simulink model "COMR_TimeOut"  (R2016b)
settings: Solver=FixedStepDiscrete  StartTime=0.0  StopTime=10.0  FixedStep=0.01  RelTol=1e-3  EnableMultiTasking=on
undefined symbols (not defined in the file or in its folder): bin2dec, COMR_cntObcTmtDiag_CW, COMR_cntVcu2A3TmtDiag_CW, COMR_flgTmtCAB_C, COMR_numPackVcuMsg_C, COMR_tiBusoffDiagEna_C, COMR_tiCabMsgTmt_C, COMR_tiCSCMsgTmt_C, COMR_tiGWMsg050Tmt_C, COMR_tiGWMsgTmt_C, COMR_tiHv638MsgTmt_C, COMR_tiMcuMsgTmt_C, COMR_tiObcMsgTmt_C, COMR_tiPackVcuMsgTmt_C, COMR_tiPwrupDiagEna_C, COMR_tiTmtBase_C, COMR_tiVcuMsgTmt_C, COMR_UAESFltDiagDisbl_C
libraries: simulink x167
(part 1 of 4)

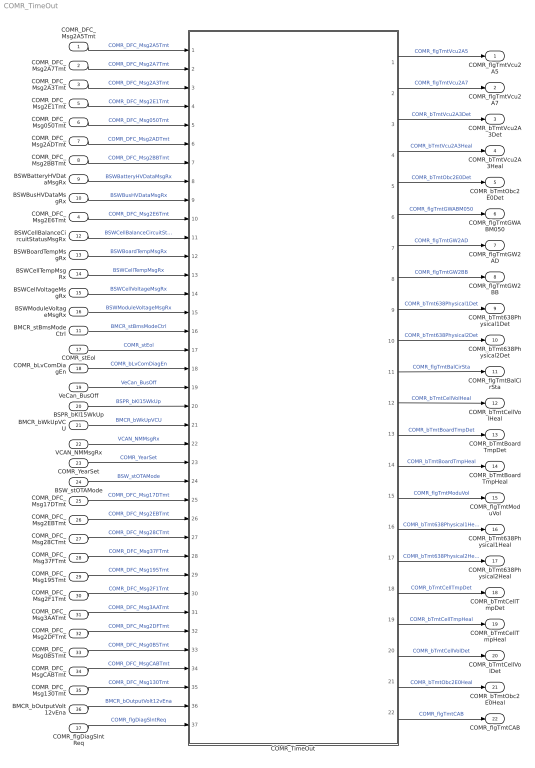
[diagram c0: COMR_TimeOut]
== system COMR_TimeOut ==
  COMR_DFC_Msg2A5Tmt : Inport
  COMR_DFC_Msg2A7Tmt : Inport  Port=2
  COMR_DFC_Msg2A3Tmt : Inport  Port=3
  COMR_DFC_Msg2E6Tmt : Inport  Port=4
  COMR_DFC_Msg2E1Tmt : Inport  Port=5
  COMR_DFC_Msg050Tmt : Inport  Port=6
  COMR_DFC_Msg2ADTmt : Inport  Port=7
  COMR_DFC_Msg2BBTmt : Inport  Port=8
  BSWBatteryHVDataMsgRx : Inport  Port=9
  BSWBusHVDataMsgRx : Inport  Port=10
  BMCR_stBmsModeCtrl : Inport  Port=11
  BSWCellBalanceCircuitStatusMsgRx : Inport  Port=12
  BSWBoardTempMsgRx : Inport  Port=13
  BSWCellTempMsgRx : Inport  Port=14
  BSWCellVoltageMsgRx : Inport  Port=15
  BSWModuleVoltageMsgRx : Inport  Port=16
  COMR_stEol : Inport  Port=17  OutDataTypeStr=boolean
  COMR_bLvComDiagEn : Inport  Port=18
  VeCan_BusOff : Inport  Port=19
  BSPR_bKl15WkUp : Inport  Port=20  OutDataTypeStr=boolean
  BMCR_bWkUpVCU : Inport  Port=21
  VCAN_NMMsgRx : Inport  Port=22
  COMR_YearSet : Inport  Port=23
  BSW_stOTAMode : Inport  Port=24  OutDataTypeStr=boolean
  COMR_DFC_Msg17DTmt : Inport  Port=25
  COMR_DFC_Msg2EBTmt : Inport  Port=26
  COMR_DFC_Msg28CTmt : Inport  Port=27
  COMR_DFC_Msg37FTmt : Inport  Port=28
  COMR_DFC_Msg195Tmt : Inport  Port=29
  COMR_DFC_Msg2F1Tmt : Inport  Port=30
  COMR_DFC_Msg3AATmt : Inport  Port=31
  COMR_DFC_Msg2DFTmt : Inport  Port=32
  COMR_DFC_Msg0B5Tmt : Inport  Port=33
  COMR_DFC_MsgCABTmt : Inport  Port=34
  COMR_DFC_Msg130Tmt : Inport  Port=35
  BMCR_bOutputVolt12vEna : Inport  Port=36
  COMR_flgDiagSlntReq : Inport  Port=37  OutDataTypeStr=boolean
  COMR_TimeOut : Subsystem
  COMR_flgTmtVcu2A5 : Outport
  COMR_flgTmtVcu2A7 : Outport  Port=2
  COMR_bTmtVcu2A3Det : Outport  Port=3
  COMR_bTmtVcu2A3Heal : Outport  Port=4
  COMR_bTmtObc2E0Det : Outport  Port=5
  COMR_flgTmtGWABM050 : Outport  Port=6
  COMR_flgTmtGW2AD : Outport  Port=7
  COMR_flgTmtGW2BB : Outport  Port=8
  COMR_bTmt638Physical1Det : Outport  Port=9
  COMR_bTmt638Physical2Det : Outport  Port=10
  COMR_flgTmtBalCirSta : Outport  Port=11
  COMR_bTmtCellVolHeal : Outport  Port=12
  COMR_bTmtBoardTmpDet : Outport  Port=13
  COMR_bTmtBoardTmpHeal : Outport  Port=14
  COMR_flgTmtModuVol : Outport  Port=15
  COMR_bTmt638Physical1Heal : Outport  Port=16
  COMR_bTmt638Physical2Heal : Outport  Port=17
  COMR_bTmtCellTmpDet : Outport  Port=18
  COMR_bTmtCellTmpHeal : Outport  Port=19
  COMR_bTmtCellVolDet : Outport  Port=20
  COMR_bTmtObc2E0Heal : Outport  Port=21
  COMR_flgTmtCAB : Outport  Port=22
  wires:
  COMR_DFC_Msg2A5Tmt/1 -> COMR_TimeOut/1(COMR_DFC_Msg2A5Tmt)  "COMR_DFC_Msg2A5Tmt"
  COMR_DFC_Msg2A7Tmt/1 -> COMR_TimeOut/2(COMR_DFC_Msg2A7Tmt)  "COMR_DFC_Msg2A7Tmt"
  COMR_DFC_Msg2A3Tmt/1 -> COMR_TimeOut/3(COMR_DFC_Msg2A3Tmt)  "COMR_DFC_Msg2A3Tmt"
  COMR_DFC_Msg2E6Tmt/1 -> COMR_TimeOut/10(COMR_DFC_Msg2E6Tmt)  "COMR_DFC_Msg2E6Tmt"
  COMR_DFC_Msg2E1Tmt/1 -> COMR_TimeOut/4(COMR_DFC_Msg2E1Tmt)  "COMR_DFC_Msg2E1Tmt"
  COMR_DFC_Msg050Tmt/1 -> COMR_TimeOut/5(COMR_DFC_Msg050Tmt)  "COMR_DFC_Msg050Tmt"
  COMR_DFC_Msg2ADTmt/1 -> COMR_TimeOut/6(COMR_DFC_Msg2ADTmt)  "COMR_DFC_Msg2ADTmt"
  COMR_DFC_Msg2BBTmt/1 -> COMR_TimeOut/7(COMR_DFC_Msg2BBTmt)  "COMR_DFC_Msg2BBTmt"
  BSWBatteryHVDataMsgRx/1 -> COMR_TimeOut/8(BSWBatteryHVDataMsgRx)  "BSWBatteryHVDataMsgRx"
  BSWBusHVDataMsgRx/1 -> COMR_TimeOut/9(BSWBusHVDataMsgRx)  "BSWBusHVDataMsgRx"
  COMR_TimeOut/1(COMR_flgTmtVcu2A5) -> COMR_flgTmtVcu2A5/1  "COMR_flgTmtVcu2A5"
  COMR_TimeOut/2(COMR_flgTmtVcu2A7) -> COMR_flgTmtVcu2A7/1  "COMR_flgTmtVcu2A7"
  COMR_TimeOut/3(COMR_bTmtVcu2A3Det) -> COMR_bTmtVcu2A3Det/1  "COMR_bTmtVcu2A3Det"
  COMR_TimeOut/4(COMR_bTmtVcu2A3Heal) -> COMR_bTmtVcu2A3Heal/1  "COMR_bTmtVcu2A3Heal"
  COMR_TimeOut/5(COMR_bTmtObc2E0Det) -> COMR_bTmtObc2E0Det/1  "COMR_bTmtObc2E0Det"
  COMR_TimeOut/6(COMR_flgTmtGWABM050) -> COMR_flgTmtGWABM050/1  "COMR_flgTmtGWABM050"
  COMR_TimeOut/7(COMR_flgTmtGW2AD) -> COMR_flgTmtGW2AD/1  "COMR_flgTmtGW2AD"
  COMR_TimeOut/8(COMR_flgTmtGW2BB) -> COMR_flgTmtGW2BB/1  "COMR_flgTmtGW2BB"
  COMR_TimeOut/9(COMR_bTmt638Physical1Det) -> COMR_bTmt638Physical1Det/1  "COMR_bTmt638Physical1Det"
  COMR_TimeOut/10(COMR_bTmt638Physical2Det) -> COMR_bTmt638Physical2Det/1  "COMR_bTmt638Physical2Det"
  BMCR_stBmsModeCtrl/1 -> COMR_TimeOut/16(BMCR_stBmsModeCtrl)  "BMCR_stBmsModeCtrl"
  BSWCellBalanceCircuitStatusMsgRx/1 -> COMR_TimeOut/11(BSWCellBalanceCircuitStatusMsgRx)  "BSWCellBalanceCircuitStatusMsgRx"
  COMR_TimeOut/12(COMR_bTmtCellVolHeal) -> COMR_bTmtCellVolHeal/1  "COMR_bTmtCellVolHeal"
  COMR_TimeOut/11(COMR_flgTmtBalCirSta) -> COMR_flgTmtBalCirSta/1  "COMR_flgTmtBalCirSta"
  COMR_TimeOut/13(COMR_bTmtBoardTmpDet) -> COMR_bTmtBoardTmpDet/1  "COMR_bTmtBoardTmpDet"
  COMR_TimeOut/14(COMR_bTmtBoardTmpHeal) -> COMR_bTmtBoardTmpHeal/1  "COMR_bTmtBoardTmpHeal"
  COMR_TimeOut/15(COMR_flgTmtModuVol) -> COMR_flgTmtModuVol/1  "COMR_flgTmtModuVol"
  BSWBoardTempMsgRx/1 -> COMR_TimeOut/12(BSWBoardTempMsgRx)  "BSWBoardTempMsgRx"
  BSWCellTempMsgRx/1 -> COMR_TimeOut/13(BSWCellTempMsgRx)  "BSWCellTempMsgRx"
  BSWCellVoltageMsgRx/1 -> COMR_TimeOut/14(BSWCellVoltageMsgRx)  "BSWCellVoltageMsgRx"
  BSWModuleVoltageMsgRx/1 -> COMR_TimeOut/15(BSWModuleVoltageMsgRx)  "BSWModuleVoltageMsgRx"
  COMR_TimeOut/16(COMR_bTmt638Physical1Heal) -> COMR_bTmt638Physical1Heal/1  "COMR_bTmt638Physical1Heal"
  COMR_TimeOut/17(COMR_bTmt638Physical2Heal) -> COMR_bTmt638Physical2Heal/1  "COMR_bTmt638Physical2Heal"
  COMR_TimeOut/18(COMR_bTmtCellTmpDet) -> COMR_bTmtCellTmpDet/1  "COMR_bTmtCellTmpDet"
  COMR_TimeOut/19(COMR_bTmtCellTmpHeal) -> COMR_bTmtCellTmpHeal/1  "COMR_bTmtCellTmpHeal"
  COMR_TimeOut/20(COMR_bTmtCellVolDet) -> COMR_bTmtCellVolDet/1  "COMR_bTmtCellVolDet"
  COMR_TimeOut/21(COMR_bTmtObc2E0Heal) -> COMR_bTmtObc2E0Heal/1  "COMR_bTmtObc2E0Heal"
  COMR_stEol/1 -> COMR_TimeOut/17(COMR_stEol)  "COMR_stEol"
  COMR_bLvComDiagEn/1 -> COMR_TimeOut/18(COMR_bLvComDiagEn)  "COMR_bLvComDiagEn"
  VeCan_BusOff/1 -> COMR_TimeOut/19(VeCan_BusOff)  "VeCan_BusOff"
  BSPR_bKl15WkUp/1 -> COMR_TimeOut/20(BSPR_bKl15WkUp)  "BSPR_bKl15WkUp"
  BMCR_bWkUpVCU/1 -> COMR_TimeOut/21(BMCR_bWkUpVCU)  "BMCR_bWkUpVCU"
  VCAN_NMMsgRx/1 -> COMR_TimeOut/22(VCAN_NMMsgRx)  "VCAN_NMMsgRx"
  COMR_YearSet/1 -> COMR_TimeOut/23(COMR_YearSet)  "COMR_YearSet"
  COMR_TimeOut/22(COMR_flgTmtCAB) -> COMR_flgTmtCAB/1  "COMR_flgTmtCAB"
  BSW_stOTAMode/1 -> COMR_TimeOut/24(BSW_stOTAMode)  "BSW_stOTAMode"
  COMR_DFC_Msg17DTmt/1 -> COMR_TimeOut/25(COMR_DFC_Msg17DTmt)  "COMR_DFC_Msg17DTmt"
  COMR_DFC_Msg130Tmt/1 -> COMR_TimeOut/35(COMR_DFC_Msg130Tmt)  "COMR_DFC_Msg130Tmt"
  COMR_DFC_Msg2EBTmt/1 -> COMR_TimeOut/26(COMR_DFC_Msg2EBTmt)  "COMR_DFC_Msg2EBTmt"
  COMR_DFC_Msg28CTmt/1 -> COMR_TimeOut/27(COMR_DFC_Msg28CTmt)  "COMR_DFC_Msg28CTmt"
  COMR_DFC_Msg37FTmt/1 -> COMR_TimeOut/28(COMR_DFC_Msg37FTmt)  "COMR_DFC_Msg37FTmt"
  COMR_DFC_Msg195Tmt/1 -> COMR_TimeOut/29(COMR_DFC_Msg195Tmt)  "COMR_DFC_Msg195Tmt"
  COMR_DFC_Msg2F1Tmt/1 -> COMR_TimeOut/30(COMR_DFC_Msg2F1Tmt)  "COMR_DFC_Msg2F1Tmt"
  COMR_DFC_Msg3AATmt/1 -> COMR_TimeOut/31(COMR_DFC_Msg3AATmt)  "COMR_DFC_Msg3AATmt"
  COMR_DFC_Msg2DFTmt/1 -> COMR_TimeOut/32(COMR_DFC_Msg2DFTmt)  "COMR_DFC_Msg2DFTmt"
  COMR_DFC_Msg0B5Tmt/1 -> COMR_TimeOut/33(COMR_DFC_Msg0B5Tmt)  "COMR_DFC_Msg0B5Tmt"
  COMR_DFC_MsgCABTmt/1 -> COMR_TimeOut/34(COMR_DFC_MsgCABTmt)  "COMR_DFC_MsgCABTmt"
  BMCR_bOutputVolt12vEna/1 -> COMR_TimeOut/36(BMCR_bOutputVolt12vEna)  "BMCR_bOutputVolt12vEna"
  COMR_flgDiagSlntReq/1 -> COMR_TimeOut/37(COMR_flgDiagSlntReq)  "COMR_flgDiagSlntReq"

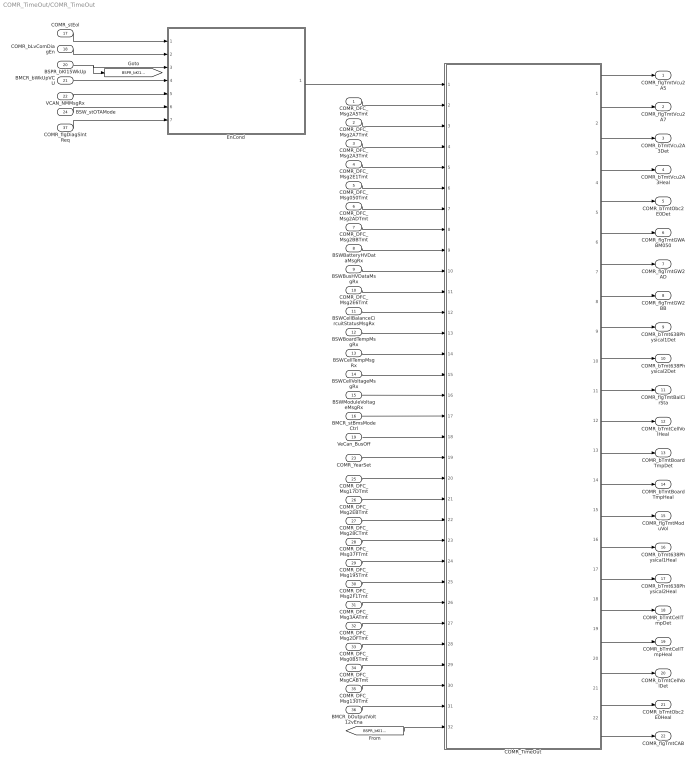
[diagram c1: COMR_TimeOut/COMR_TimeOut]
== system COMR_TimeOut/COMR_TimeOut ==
  COMR_DFC_Msg2A5Tmt : Inport
  COMR_DFC_Msg2A7Tmt : Inport  Port=2
  COMR_DFC_Msg2A3Tmt : Inport  Port=3
  COMR_DFC_Msg2E1Tmt : Inport  Port=4
  COMR_DFC_Msg050Tmt : Inport  Port=5
  COMR_DFC_Msg2ADTmt : Inport  Port=6
  COMR_DFC_Msg2BBTmt : Inport  Port=7
  BSWBatteryHVDataMsgRx : Inport  Port=8
  BSWBusHVDataMsgRx : Inport  Port=9
  COMR_DFC_Msg2E6Tmt : Inport  Port=10
  BSWCellBalanceCircuitStatusMsgRx : Inport  Port=11
  BSWBoardTempMsgRx : Inport  Port=12
  BSWCellTempMsgRx : Inport  Port=13
  BSWCellVoltageMsgRx : Inport  Port=14
  BSWModuleVoltageMsgRx : Inport  Port=15
  BMCR_stBmsModeCtrl : Inport  Port=16
  COMR_stEol : Inport  Port=17  OutDataTypeStr=boolean
  COMR_bLvComDiagEn : Inport  Port=18
  VeCan_BusOff : Inport  Port=19
  BSPR_bKl15WkUp : Inport  Port=20  OutDataTypeStr=boolean
  BMCR_bWkUpVCU : Inport  Port=21
  VCAN_NMMsgRx : Inport  Port=22
  COMR_YearSet : Inport  Port=23
  BSW_stOTAMode : Inport  Port=24  OutDataTypeStr=boolean
  COMR_DFC_Msg17DTmt : Inport  Port=25
  COMR_DFC_Msg2EBTmt : Inport  Port=26
  COMR_DFC_Msg28CTmt : Inport  Port=27
  COMR_DFC_Msg37FTmt : Inport  Port=28
  COMR_DFC_Msg195Tmt : Inport  Port=29
  COMR_DFC_Msg2F1Tmt : Inport  Port=30
  COMR_DFC_Msg3AATmt : Inport  Port=31
  COMR_DFC_Msg2DFTmt : Inport  Port=32
  COMR_DFC_Msg0B5Tmt : Inport  Port=33
  COMR_DFC_MsgCABTmt : Inport  Port=34
  COMR_DFC_Msg130Tmt : Inport  Port=35
  BMCR_bOutputVolt12vEna : Inport  Port=36
  COMR_flgDiagSlntReq : Inport  Port=37  OutDataTypeStr=boolean
  COMR_TimeOut : Subsystem
  EnCond : Subsystem
  COMR_flgTmtVcu2A5 : Outport
  COMR_flgTmtVcu2A7 : Outport  Port=2
  COMR_bTmtVcu2A3Det : Outport  Port=3
  COMR_bTmtVcu2A3Heal : Outport  Port=4
  COMR_bTmtObc2E0Det : Outport  Port=5
  COMR_flgTmtGWABM050 : Outport  Port=6
  COMR_flgTmtGW2AD : Outport  Port=7
  COMR_flgTmtGW2BB : Outport  Port=8
  COMR_bTmt638Physical1Det : Outport  Port=9
  COMR_bTmt638Physical2Det : Outport  Port=10
  COMR_flgTmtBalCirSta : Outport  Port=11
  COMR_bTmtCellVolHeal : Outport  Port=12
  COMR_bTmtBoardTmpDet : Outport  Port=13
  COMR_bTmtBoardTmpHeal : Outport  Port=14
  COMR_flgTmtModuVol : Outport  Port=15
  COMR_bTmt638Physical1Heal : Outport  Port=16
  COMR_bTmt638Physical2Heal : Outport  Port=17
  COMR_bTmtCellTmpDet : Outport  Port=18
  COMR_bTmtCellTmpHeal : Outport  Port=19
  COMR_bTmtCellVolDet : Outport  Port=20
  COMR_bTmtObc2E0Heal : Outport  Port=21
  COMR_flgTmtCAB : Outport  Port=22
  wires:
  COMR_DFC_Msg2A5Tmt/1 -> COMR_TimeOut/2(COMR_DFC_Msg2A5Tmt)
  COMR_DFC_Msg2A7Tmt/1 -> COMR_TimeOut/3(COMR_DFC_Msg2A7Tmt)
  COMR_DFC_Msg2A3Tmt/1 -> COMR_TimeOut/4(COMR_DFC_Msg2A3Tmt)
  COMR_DFC_Msg2E1Tmt/1 -> COMR_TimeOut/5(COMR_DFC_Msg2E1Tmt)
  COMR_DFC_Msg050Tmt/1 -> COMR_TimeOut/6(COMR_DFC_Msg050Tmt)
  COMR_DFC_Msg2ADTmt/1 -> COMR_TimeOut/7(COMR_DFC_Msg2ADTmt)
  COMR_DFC_Msg2BBTmt/1 -> COMR_TimeOut/8(COMR_DFC_Msg2BBTmt)
  BSWBatteryHVDataMsgRx/1 -> COMR_TimeOut/9(BSWBatteryHVDataMsgRx)
  BSWBusHVDataMsgRx/1 -> COMR_TimeOut/10(BSWBusHVDataMsgRx)
  COMR_DFC_Msg2E6Tmt/1 -> COMR_TimeOut/11(COMR_DFC_Msg2E6Tmt)
  BSWCellBalanceCircuitStatusMsgRx/1 -> COMR_TimeOut/12(BSWCellBalanceCircuitStatusMsgRx)
  BSWBoardTempMsgRx/1 -> COMR_TimeOut/13(BSWBoardTempMsgRx)
  BSWCellTempMsgRx/1 -> COMR_TimeOut/14(BSWCellTempMsgRx)
  BSWCellVoltageMsgRx/1 -> COMR_TimeOut/15(BSWCellVoltageMsgRx)
  BSWModuleVoltageMsgRx/1 -> COMR_TimeOut/16(BSWModuleVoltageMsgRx)
  BMCR_stBmsModeCtrl/1 -> COMR_TimeOut/17(BMCR_stBmsModeCtrl)
  COMR_TimeOut/1(COMR_flgTmtVcu2A5) -> COMR_flgTmtVcu2A5/1
  COMR_TimeOut/2(COMR_flgTmtVcu2A7) -> COMR_flgTmtVcu2A7/1
  COMR_TimeOut/3(COMR_bTmtVcu2A3Det) -> COMR_bTmtVcu2A3Det/1
  COMR_TimeOut/4(COMR_bTmtVcu2A3Heal) -> COMR_bTmtVcu2A3Heal/1
  COMR_TimeOut/5(COMR_bTmtObc2E0Det) -> COMR_bTmtObc2E0Det/1
  COMR_TimeOut/6(COMR_flgTmtGWABM050) -> COMR_flgTmtGWABM050/1
  COMR_TimeOut/7(COMR_flgTmtGW2AD) -> COMR_flgTmtGW2AD/1
  COMR_TimeOut/8(COMR_flgTmtGW2BB) -> COMR_flgTmtGW2BB/1
  COMR_TimeOut/9(COMR_bTmt638Physical1Det) -> COMR_bTmt638Physical1Det/1
  COMR_TimeOut/10(COMR_bTmt638Physical2Det) -> COMR_bTmt638Physical2Det/1
  COMR_TimeOut/11(COMR_flgTmtBalCirSta) -> COMR_flgTmtBalCirSta/1
  COMR_TimeOut/12(COMR_bTmtCellVolHeal) -> COMR_bTmtCellVolHeal/1
  COMR_TimeOut/13(COMR_bTmtBoardTmpDet) -> COMR_bTmtBoardTmpDet/1
  COMR_TimeOut/14(COMR_bTmtBoardTmpHeal) -> COMR_bTmtBoardTmpHeal/1
  COMR_TimeOut/15(COMR_flgTmtModuVol) -> COMR_flgTmtModuVol/1
  COMR_TimeOut/16(COMR_bTmt638Physical1Heal) -> COMR_bTmt638Physical1Heal/1
  COMR_TimeOut/17(COMR_bTmt638Physical2Heal) -> COMR_bTmt638Physical2Heal/1
  COMR_TimeOut/18(COMR_bTmtCellTmpDet) -> COMR_bTmtCellTmpDet/1
  COMR_TimeOut/19(COMR_bTmtCellTmpHeal) -> COMR_bTmtCellTmpHeal/1
  COMR_TimeOut/20(COMR_bTmtCellVolDet) -> COMR_bTmtCellVolDet/1
  COMR_TimeOut/21(COMR_bTmtObc2E0Heal) -> COMR_bTmtObc2E0Heal/1
  COMR_stEol/1 -> EnCond/1(COMR_stEol)
  EnCond/1(COMR_bTiOutChkEn) -> COMR_TimeOut/1(COMR_bTiOutChkEn)
  COMR_bLvComDiagEn/1 -> EnCond/2(COMR_bLvComDiagEn)
  VeCan_BusOff/1 -> COMR_TimeOut/18(VeCan_BusOff)
  BSPR_bKl15WkUp/1 -> EnCond/3(BSPR_bKl15WkUp), [BSPR_bKl15WkUp]
  BMCR_bWkUpVCU/1 -> EnCond/4(BMCR_bWkUpVCU)
  VCAN_NMMsgRx/1 -> EnCond/5(VCAN_NMMsgRx)
  COMR_YearSet/1 -> COMR_TimeOut/19(COMR_YearSet)
  COMR_TimeOut/22(COMR_flgTmtCAB) -> COMR_flgTmtCAB/1
  BSW_stOTAMode/1 -> EnCond/6(BSW_stOTAMode)
  COMR_DFC_Msg17DTmt/1 -> COMR_TimeOut/20(COMR_DFC_Msg17DTmt)
  COMR_DFC_Msg130Tmt/1 -> COMR_TimeOut/30(COMR_DFC_Msg130Tmt)
  COMR_DFC_Msg2EBTmt/1 -> COMR_TimeOut/21(COMR_DFC_Msg2EBTmt)
  COMR_DFC_Msg28CTmt/1 -> COMR_TimeOut/22(COMR_DFC_Msg28CTmt)
  COMR_DFC_Msg37FTmt/1 -> COMR_TimeOut/23(COMR_DFC_Msg37FTmt)
  COMR_DFC_Msg195Tmt/1 -> COMR_TimeOut/24(COMR_DFC_Msg195Tmt)
  COMR_DFC_Msg2F1Tmt/1 -> COMR_TimeOut/25(COMR_DFC_Msg2F1Tmt)
  COMR_DFC_Msg3AATmt/1 -> COMR_TimeOut/26(COMR_DFC_Msg3AATmt)
  COMR_DFC_Msg2DFTmt/1 -> COMR_TimeOut/27(COMR_DFC_Msg2DFTmt)
  COMR_DFC_Msg0B5Tmt/1 -> COMR_TimeOut/28(COMR_DFC_Msg0B5Tmt)
  COMR_DFC_MsgCABTmt/1 -> COMR_TimeOut/29(COMR_DFC_MsgCABTmt)
  BMCR_bOutputVolt12vEna/1 -> COMR_TimeOut/31(BMCR_bOutputVolt12vEna)
  COMR_flgDiagSlntReq/1 -> EnCond/7(COMR_flgDiagSlntReq)
  [BSPR_bKl15WkUp] -> COMR_TimeOut/32(BSPR_bKl15WkUp)

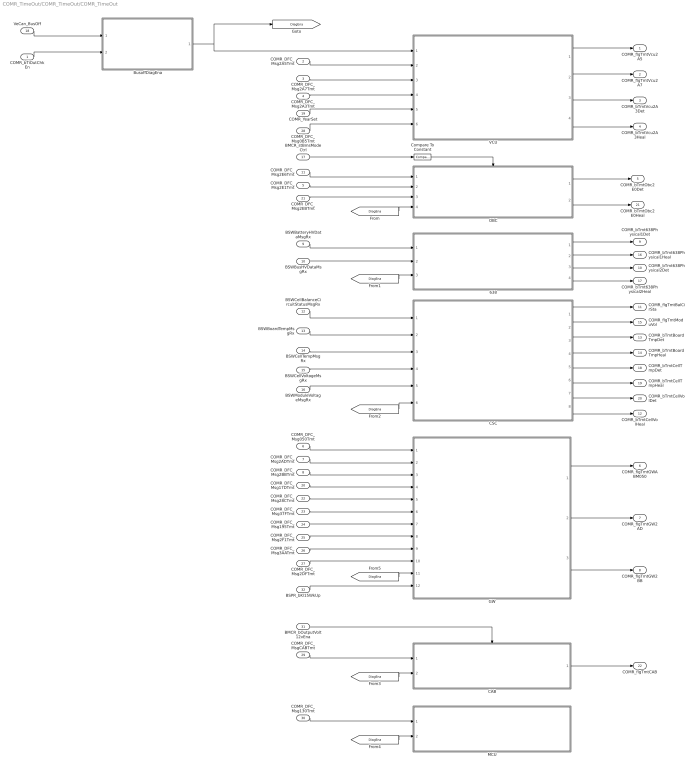
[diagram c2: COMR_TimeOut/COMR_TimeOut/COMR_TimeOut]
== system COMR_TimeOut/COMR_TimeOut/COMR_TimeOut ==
  COMR_bTiOutChkEn : Inport
  COMR_DFC_Msg2A5Tmt : Inport  Port=2
  COMR_DFC_Msg2A7Tmt : Inport  Port=3
  COMR_DFC_Msg2A3Tmt : Inport  Port=4
  COMR_DFC_Msg2E1Tmt : Inport  Port=5
  COMR_DFC_Msg050Tmt : Inport  Port=6
  COMR_DFC_Msg2ADTmt : Inport  Port=7
  COMR_DFC_Msg2BBTmt : Inport  Port=8
  BSWBatteryHVDataMsgRx : Inport  Port=9
  BSWBusHVDataMsgRx : Inport  Port=10
  COMR_DFC_Msg2E6Tmt : Inport  Port=11
  BSWCellBalanceCircuitStatusMsgRx : Inport  Port=12
  BSWBoardTempMsgRx : Inport  Port=13
  BSWCellTempMsgRx : Inport  Port=14
  BSWCellVoltageMsgRx : Inport  Port=15
  BSWModuleVoltageMsgRx : Inport  Port=16
  BMCR_stBmsModeCtrl : Inport  Port=17
  VeCan_BusOff : Inport  Port=18
  COMR_YearSet : Inport  Port=19
  COMR_DFC_Msg17DTmt : Inport  Port=20
  COMR_DFC_Msg2EBTmt : Inport  Port=21
  COMR_DFC_Msg28CTmt : Inport  Port=22
  COMR_DFC_Msg37FTmt : Inport  Port=23
  COMR_DFC_Msg195Tmt : Inport  Port=24
  COMR_DFC_Msg2F1Tmt : Inport  Port=25
  COMR_DFC_Msg3AATmt : Inport  Port=26
  COMR_DFC_Msg2DFTmt : Inport  Port=27
  COMR_DFC_Msg0B5Tmt : Inport  Port=28
  COMR_DFC_MsgCABTmt : Inport  Port=29
  COMR_DFC_Msg130Tmt : Inport  Port=30
  BMCR_bOutputVolt12vEna : Inport  Port=31
  BSPR_bKl15WkUp : Inport  Port=32  OutDataTypeStr=boolean
  638 : Subsystem
  BusoffDiagEna : Subsystem
  CAB : Subsystem
  CSC : Subsystem
  Compare To Constant : simulink/Logic and Bit Operations/Compare To Constant  relop===  const=6  OutDataTypeStr=boolean
  GW : Subsystem
  MCU : Subsystem
  OBC : Subsystem
  VCU : Subsystem
  COMR_flgTmtVcu2A5 : Outport  InitialOutput=[0]
  COMR_flgTmtVcu2A7 : Outport  Port=2  InitialOutput=[0]
  COMR_bTmtVcu2A3Det : Outport  Port=3  InitialOutput=[0]
  COMR_bTmtVcu2A3Heal : Outport  Port=4  InitialOutput=[0]
  COMR_bTmtObc2E0Det : Outport  Port=5  InitialOutput=[0]
  COMR_flgTmtGWABM050 : Outport  Port=6
  COMR_flgTmtGW2AD : Outport  Port=7
  COMR_flgTmtGW2BB : Outport  Port=8
  COMR_bTmt638Physical1Det : Outport  Port=9  InitialOutput=[0]
  COMR_bTmt638Physical2Det : Outport  Port=10
  COMR_flgTmtBalCirSta : Outport  Port=11  InitialOutput=[0]
  COMR_bTmtCellVolHeal : Outport  Port=12
  COMR_bTmtBoardTmpDet : Outport  Port=13
  COMR_bTmtBoardTmpHeal : Outport  Port=14
  COMR_flgTmtModuVol : Outport  Port=15  InitialOutput=[0]
  COMR_bTmt638Physical1Heal : Outport  Port=16
  COMR_bTmt638Physical2Heal : Outport  Port=17
  COMR_bTmtCellTmpDet : Outport  Port=18
  COMR_bTmtCellTmpHeal : Outport  Port=19
  COMR_bTmtCellVolDet : Outport  Port=20
  COMR_bTmtObc2E0Heal : Outport  Port=21  InitialOutput=[0]
  COMR_flgTmtCAB : Outport  Port=22
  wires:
  BSWBoardTempMsgRx/1 -> CSC/2(BSWBoardTempMsgRx)
  COMR_DFC_Msg2A3Tmt/1 -> VCU/4(COMR_DFC_Msg2A3Tmt)
  COMR_DFC_Msg2A7Tmt/1 -> VCU/3(COMR_DFC_Msg2A7Tmt)
  638/4(COMR_bTmt638Physical2Heal) -> COMR_bTmt638Physical2Heal/1
  COMR_DFC_Msg2A5Tmt/1 -> VCU/2(COMR_DFC_Msg2A5Tmt)
  CSC/2(COMR_flgTmtModuVol) -> COMR_flgTmtModuVol/1
  CSC/3(COMR_bTmtBoardTmpDet) -> COMR_bTmtBoardTmpDet/1
  CSC/4(COMR_bTmtBoardTmpHeal) -> COMR_bTmtBoardTmpHeal/1
  CSC/8(COMR_bTmtCellVolHeal) -> COMR_bTmtCellVolHeal/1
  BSWCellBalanceCircuitStatusMsgRx/1 -> CSC/1(BSWCellBalanceCircuitStatusMsgRx)
  CSC/1(COMR_flgTmtBalCirSta) -> COMR_flgTmtBalCirSta/1
  638/3(COMR_bTmt638Physical2Det) -> COMR_bTmt638Physical2Det/1
  BSWBusHVDataMsgRx/1 -> 638/2(BSWBusHVDataMsgRx)
  638/1(COMR_bTmt638Physical1Det) -> COMR_bTmt638Physical1Det/1
  BSWBatteryHVDataMsgRx/1 -> 638/1(BSWBatteryHVDataMsgRx)
  GW/2(COMR_flgTmtGW2AD) -> COMR_flgTmtGW2AD/1
  GW/3(COMR_flgTmtGW2BB) -> COMR_flgTmtGW2BB/1
  GW/1(COMR_flgTmtGWABM050) -> COMR_flgTmtGWABM050/1
  COMR_DFC_Msg2ADTmt/1 -> GW/2(COMR_DFC_Msg2ADTmt)
  COMR_DFC_Msg2BBTmt/1 -> GW/3(COMR_DFC_Msg2BBTmt)
  638/2(COMR_bTmt638Physical1Heal) -> COMR_bTmt638Physical1Heal/1
  BMCR_stBmsModeCtrl/1 -> Compare To Constant/1
  BSWModuleVoltageMsgRx/1 -> CSC/5(BSWModuleVoltageMsgRx)
  BSWCellTempMsgRx/1 -> CSC/3(BSWCellTempMsgRx)
  BSWCellVoltageMsgRx/1 -> CSC/4(BSWCellVoltageMsgRx)
  OBC/1(COMR_bTmtObc2E6Det) -> COMR_bTmtObc2E0Det/1
  COMR_DFC_Msg050Tmt/1 -> GW/1(COMR_DFC_Msg050Tmt)
  COMR_DFC_Msg2E6Tmt/1 -> OBC/1(COMR_DFC_Msg2E6Tmt)
  VCU/4(COMR_bTmtVcu2A3Heal) -> COMR_bTmtVcu2A3Heal/1
  VCU/3(COMR_bTmtVcu2A3Det) -> COMR_bTmtVcu2A3Det/1
  COMR_DFC_Msg2E1Tmt/1 -> OBC/2(COMR_DFC_Msg2E1Tmt)
  VCU/1(COMR_flgTmtVcu2A5) -> COMR_flgTmtVcu2A5/1
  VCU/2(COMR_flgTmtVcu2A7) -> COMR_flgTmtVcu2A7/1
  CSC/5(COMR_bTmtCellTmpDet) -> COMR_bTmtCellTmpDet/1
  OBC/2(COMR_bTmtObc2E6Heal) -> COMR_bTmtObc2E0Heal/1
  CSC/7(COMR_bTmtCellVolDet) -> COMR_bTmtCellVolDet/1
  CSC/6(COMR_bTmtCellTmpHeal) -> COMR_bTmtCellTmpHeal/1
  Compare To Constant/1 -> OBC/Enable
  [DiagEna] -> OBC/4(DiagEna)
  [DiagEna] -> 638/3(DiagEna)
  [DiagEna] -> CSC/6(DiagEna)
  VeCan_BusOff/1 -> BusoffDiagEna/1(VeCan_BusOff)
  BusoffDiagEna/1(DiagEna) -> [DiagEna], VCU/1(DiagEna)
  COMR_YearSet/1 -> VCU/5(COMR_YearSet)
  CAB/1(COMR_flgTmtCAB) -> COMR_flgTmtCAB/1
  COMR_DFC_Msg0B5Tmt/1 -> VCU/6(COMR_DFC_Msg0B5Tmt)
  COMR_DFC_Msg2EBTmt/1 -> OBC/3(COMR_DFC_Msg2EBTmt)
  COMR_DFC_MsgCABTmt/1 -> CAB/1(COMR_DFC_MsgCABTmt)
  [DiagEna] -> CAB/2(DiagEna)
  [DiagEna] -> MCU/2(DiagEna)
  COMR_DFC_Msg130Tmt/1 -> MCU/1(COMR_DFC_Msg130Tmt)
  COMR_DFC_Msg17DTmt/1 -> GW/4(COMR_DFC_Msg17DTmt)
  COMR_DFC_Msg28CTmt/1 -> GW/5(COMR_DFC_Msg28CTmt)
  COMR_DFC_Msg37FTmt/1 -> GW/6(COMR_DFC_Msg37FTmt)
  COMR_DFC_Msg195Tmt/1 -> GW/7(COMR_DFC_Msg195Tmt)
  COMR_DFC_Msg2F1Tmt/1 -> GW/8(COMR_DFC_Msg2F1Tmt)
  COMR_DFC_Msg3AATmt/1 -> GW/9(COMR_DFC_Msg3AATmt)
  COMR_DFC_Msg2DFTmt/1 -> GW/10(COMR_DFC_Msg2DFTmt)
  [DiagEna] -> GW/11(DiagEna)
  BMCR_bOutputVolt12vEna/1 -> CAB/Enable
  COMR_bTiOutChkEn/1 -> BusoffDiagEna/2(COMR_bTiOutChkEn)
  BSPR_bKl15WkUp/1 -> GW/12(BSPR_bKl15WkUp)

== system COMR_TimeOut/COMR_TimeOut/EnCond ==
  COMR_stEol : Inport  OutDataTypeStr=boolean
  COMR_bLvComDiagEn : Inport  Port=2
  BSPR_bKl15WkUp : Inport  Port=3  OutDataTypeStr=boolean
  BMCR_bWkUpVCU : Inport  Port=4
  VCAN_NMMsgRx : Inport  Port=5
  BSW_stOTAMode : Inport  Port=6  OutDataTypeStr=boolean
  COMR_flgDiagSlntReq : Inport  Port=7  OutDataTypeStr=boolean
  Constant1 : Constant  Value=COMR_tiPwrupDiagEna_C
  Logical Operator : Logic  AllPortsSameDT=off  OutDataTypeStr=boolean
  Logical Operator1 : Logic  Operator=OR  Inputs=3  AllPortsSameDT=off  OutDataTypeStr=boolean
  Logical Operator2 : Logic  Operator=NOT  AllPortsSameDT=off  OutDataTypeStr=boolean
  Logical Operator3 : Logic  Inputs=4  AllPortsSameDT=off  OutDataTypeStr=boolean
  Logical Operator4 : Logic  Operator=NOT  AllPortsSameDT=off  OutDataTypeStr=boolean
  Logical Operator5 : Logic  Operator=NOT  AllPortsSameDT=off  OutDataTypeStr=boolean
  TONV_10msTimeDebounce : Subsystem  TreatAsAtomicUnit=on  RTWFcnName=TONV_10msTimeDebounce  RTWFileName=SrvLib
  COMR_bTiOutChkEn : Outport
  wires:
  Constant1/1 -> TONV_10msTimeDebounce/2(T)
  Logical Operator/1 -> COMR_bTiOutChkEn/1  "COMR_bTiOutChkEn"
  COMR_stEol/1 -> Logical Operator2/1
  TONV_10msTimeDebounce/1(y) -> Logical Operator/1
  COMR_bLvComDiagEn/1 -> Logical Operator/2
  BSPR_bKl15WkUp/1 -> Logical Operator1/1
  BMCR_bWkUpVCU/1 -> Logical Operator1/2
  VCAN_NMMsgRx/1 -> Logical Operator1/3
  Logical Operator2/1 -> Logical Operator3/2
  Logical Operator1/1 -> Logical Operator3/1
  Logical Operator3/1 -> TONV_10msTimeDebounce/1(u)
  Logical Operator4/1 -> Logical Operator3/3
  BSW_stOTAMode/1 -> Logical Operator4/1
  COMR_flgDiagSlntReq/1 -> Logical Operator5/1
  Logical Operator5/1 -> Logical Operator3/4

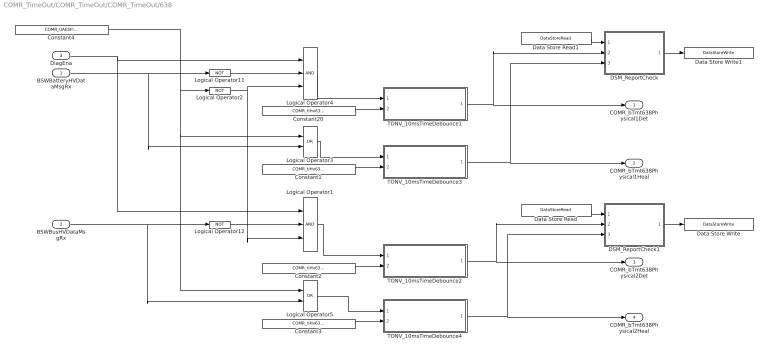
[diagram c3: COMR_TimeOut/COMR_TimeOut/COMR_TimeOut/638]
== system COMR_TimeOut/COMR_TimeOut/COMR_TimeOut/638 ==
  BSWBatteryHVDataMsgRx : Inport
  BSWBusHVDataMsgRx : Inport  Port=2
  DiagEna : Inport  Port=3
  Constant{1..3,20} (4 alike) : Constant  Value=COMR_tiHv638MsgTmt_C
  Constant4 : Constant  Value=COMR_UAESFltDiagDisbl_C
  DSM_ReportCheck : Subsystem  TreatAsAtomicUnit=on  RTWFcnName=DSM_ReportCheck  RTWFileName=SrvLib
  DSM_ReportCheck1 : Subsystem  TreatAsAtomicUnit=on  RTWFcnName=DSM_ReportCheck  RTWFileName=SrvLib
  Data Store Read : DataStoreRead  DataStoreName=DFC_BusHVMsgTmt
  Data Store Read1 : DataStoreRead  DataStoreName=DFC_BattHVMsgTmt
  Data Store Write : DataStoreWrite  DataStoreName=DFC_BusHVMsgTmt
  Data Store Write1 : DataStoreWrite  DataStoreName=DFC_BattHVMsgTmt
  Logical Operator1 : Logic  Inputs=3  AllPortsSameDT=off  OutDataTypeStr=boolean
  Logical Operator11 : Logic  Operator=NOT  AllPortsSameDT=off  OutDataTypeStr=boolean
  Logical Operator12 : Logic  Operator=NOT  AllPortsSameDT=off  OutDataTypeStr=boolean
  Logical Operator2 : Logic  Operator=NOT  AllPortsSameDT=off  OutDataTypeStr=boolean
  Logical Operator3 : Logic  Operator=OR  AllPortsSameDT=off  OutDataTypeStr=boolean
  Logical Operator4 : Logic  Inputs=3  AllPortsSameDT=off  OutDataTypeStr=boolean
  Logical Operator5 : Logic  Operator=OR  AllPortsSameDT=off  OutDataTypeStr=boolean
  TONV_10msTimeDebounce1 : Subsystem  TreatAsAtomicUnit=on  RTWFcnName=TONV_10msTimeDebounce  RTWFileName=SrvLib
  TONV_10msTimeDebounce2 : Subsystem  TreatAsAtomicUnit=on  RTWFcnName=TONV_10msTimeDebounce  RTWFileName=SrvLib
  TONV_10msTimeDebounce3 : Subsystem  TreatAsAtomicUnit=on  RTWFcnName=TONV_10msTimeDebounce  RTWFileName=SrvLib
  TONV_10msTimeDebounce4 : Subsystem  TreatAsAtomicUnit=on  RTWFcnName=TONV_10msTimeDebounce  RTWFileName=SrvLib
  COMR_bTmt638Physical1Det : Outport  InitialOutput=[0]
  COMR_bTmt638Physical1Heal : Outport  Port=2  InitialOutput=[0]
  COMR_bTmt638Physical2Det : Outport  Port=3  InitialOutput=[0]
  COMR_bTmt638Physical2Heal : Outport  Port=4  InitialOutput=[0]
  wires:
  TONV_10msTimeDebounce1/1(y) -> DSM_ReportCheck/2(Err), COMR_bTmt638Physical1Det/1
  Constant2/1 -> TONV_10msTimeDebounce2/2(T)
  Logical Operator11/1 -> Logical Operator4/2
  Constant20/1 -> TONV_10msTimeDebounce1/2(T)
  TONV_10msTimeDebounce3/1(y) -> DSM_ReportCheck/3(Heal), COMR_bTmt638Physical1Heal/1
  Constant1/1 -> TONV_10msTimeDebounce3/2(T)
  Constant3/1 -> TONV_10msTimeDebounce4/2(T)
  TONV_10msTimeDebounce2/1(y) -> DSM_ReportCheck1/2(Err), COMR_bTmt638Physical2Det/1
  TONV_10msTimeDebounce4/1(y) -> DSM_ReportCheck1/3(Heal), COMR_bTmt638Physical2Heal/1
  DSM_ReportCheck1/1(Dfc_id) -> Data Store Write/1
  Data Store Read/1 -> DSM_ReportCheck1/1(Dfc_id_nv)
  Data Store Read1/1 -> DSM_ReportCheck/1(Dfc_id_nv)
  DSM_ReportCheck/1(Dfc_id) -> Data Store Write1/1
  BSWBatteryHVDataMsgRx/1 -> Logical Operator3/2, Logical Operator11/1
  BSWBusHVDataMsgRx/1 -> Logical Operator12/1, Logical Operator5/2
  DiagEna/1 -> Logical Operator4/1, Logical Operator1/1
  Logical Operator1/1 -> TONV_10msTimeDebounce2/1(u)
  Logical Operator4/1 -> TONV_10msTimeDebounce1/1(u)
  Logical Operator12/1 -> Logical Operator1/2
  Constant4/1 -> Logical Operator5/1, Logical Operator3/1, Logical Operator2/1
  Logical Operator2/1 -> Logical Operator4/3, Logical Operator1/3
  Logical Operator3/1 -> TONV_10msTimeDebounce3/1(u)
  Logical Operator5/1 -> TONV_10msTimeDebounce4/1(u)

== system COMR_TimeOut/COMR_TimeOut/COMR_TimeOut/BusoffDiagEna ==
  VeCan_BusOff : Inport
  COMR_bTiOutChkEn : Inport  Port=2
  Constant10 : Constant  Value=COMR_UAESFltDiagDisbl_C
  Constant8 : Constant  Value=0  OutDataTypeStr=boolean
  EdgeFalling : Subsystem  TreatAsAtomicUnit=on  RTWFcnName=EdgeFalling  RTWFileName=SrvLib
  Logical Operator : Logic  Operator=NOT  AllPortsSameDT=off  OutDataTypeStr=boolean
  Logical Operator1 : Logic  AllPortsSameDT=off  OutDataTypeStr=boolean
  Logical Operator2 : Logic  AllPortsSameDT=off  OutDataTypeStr=boolean
  StateRetention2 : Subsystem
  Switch : Switch  Criteria=u2 ~= 0
  DiagEna : Outport
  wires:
  VeCan_BusOff/1 -> EdgeFalling/1(u), Logical Operator/1
  StateRetention2/1(_Out) -> Logical Operator1/1
  EdgeFalling/1(y) -> StateRetention2/1(u)
  Constant8/1 -> StateRetention2/2(clc)
  Logical Operator/1 -> Logical Operator1/2
  Logical Operator1/1 -> Switch/3
  Constant10/1 -> Switch/1, Switch/2
  Switch/1 -> Logical Operator2/1
  Logical Operator2/1 -> DiagEna/1
  COMR_bTiOutChkEn/1 -> Logical Operator2/2

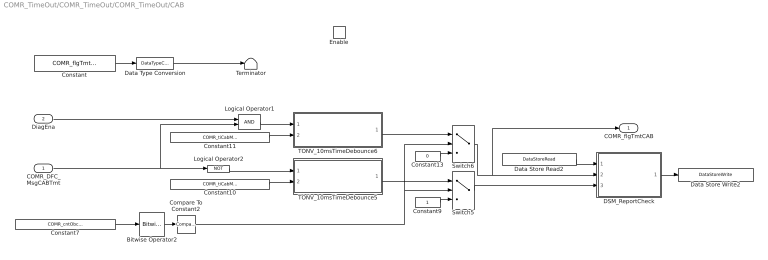
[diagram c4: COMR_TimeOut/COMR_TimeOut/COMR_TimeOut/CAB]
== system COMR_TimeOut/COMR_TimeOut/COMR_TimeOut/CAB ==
  COMR_DFC_MsgCABTmt : Inport
  DiagEna : Inport  Port=2
  Enable : EnablePort  StatesWhenEnabling=reset
  Bitwise Operator2 : simulink/Logic and Bit Operations/Bitwise Operator  logicop=AND  UseBitMask=on  BitMask=bin2dec('00010000')  BitMaskRealWorld=Stored Integer
  Compare To Constant2 : simulink/Logic and Bit Operations/Compare To Constant  relop===  const=16  OutDataTypeStr=boolean
  Constant : Constant  Value=COMR_flgTmtCAB_C
  Constant10 : Constant  Value=COMR_tiCabMsgTmt_C
  Constant11 : Constant  Value=COMR_tiCabMsgTmt_C
  Constant13 : Constant  Value=0  OutDataTypeStr=boolean
  Constant7 : Constant  Value=COMR_cntObcTmtDiag_CW
  Constant9 : Constant  OutDataTypeStr=boolean
  DSM_ReportCheck : Subsystem  TreatAsAtomicUnit=on  RTWFcnName=DSM_ReportCheck  RTWFileName=SrvLib
  Data Store Read2 : DataStoreRead  DataStoreName=DFC_MsgCABTmt
  Data Store Write2 : DataStoreWrite  DataStoreName=DFC_MsgCABTmt
  Data Type Conversion : DataTypeConversion  OutDataTypeStr=boolean
  Logical Operator1 : Logic  AllPortsSameDT=off  OutDataTypeStr=boolean
  Logical Operator2 : Logic  Operator=NOT  AllPortsSameDT=off  OutDataTypeStr=boolean
  Switch5 : Switch  Criteria=u2 > Threshold
  Switch6 : Switch  Criteria=u2 > Threshold
  TONV_10msTimeDebounce5 : Subsystem  TreatAsAtomicUnit=on  RTWFcnName=TONV_10msTimeDebounce  RTWFileName=SrvLib
  TONV_10msTimeDebounce6 : Subsystem  TreatAsAtomicUnit=on  RTWFcnName=TONV_10msTimeDebounce  RTWFileName=SrvLib
  Terminator : Terminator
  COMR_flgTmtCAB : Outport
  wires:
  Constant/1 -> Data Type Conversion/1
  Data Type Conversion/1 -> Terminator/1
  Compare To Constant2/1 -> Switch5/2, Switch6/2
  Constant7/1 -> Bitwise Operator2/1
  Bitwise Operator2/1 -> Compare To Constant2/1
  DiagEna/1 -> Logical Operator1/1
  Constant11/1 -> TONV_10msTimeDebounce6/2(T)
  DSM_ReportCheck/1(Dfc_id) -> Data Store Write2/1
  Constant10/1 -> TONV_10msTimeDebounce5/2(T)
  Constant13/1 -> Switch6/3
  Constant9/1 -> Switch5/3
  TONV_10msTimeDebounce6/1(y) -> Switch6/1
  TONV_10msTimeDebounce5/1(y) -> Switch5/1
  Switch5/1 -> DSM_ReportCheck/3(Heal)
  Data Store Read2/1 -> DSM_ReportCheck/1(Dfc_id_nv)
  Switch6/1 -> DSM_ReportCheck/2(Err), COMR_flgTmtCAB/1
  COMR_DFC_MsgCABTmt/1 -> Logical Operator1/2, Logical Operator2/1
  Logical Operator1/1 -> TONV_10msTimeDebounce6/1(u)
  Logical Operator2/1 -> TONV_10msTimeDebounce5/1(u)

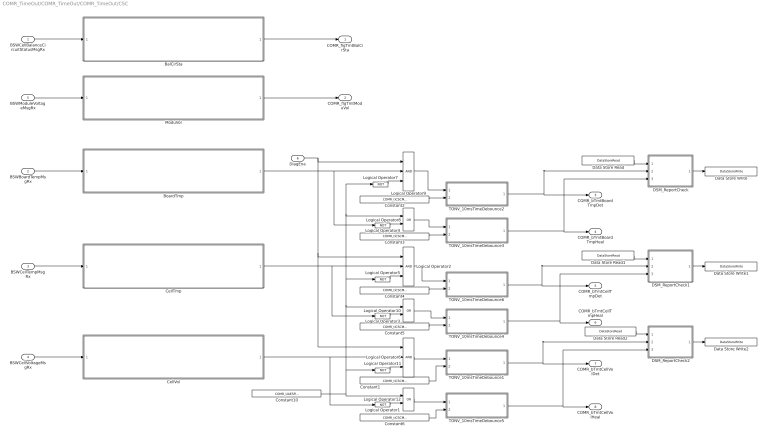
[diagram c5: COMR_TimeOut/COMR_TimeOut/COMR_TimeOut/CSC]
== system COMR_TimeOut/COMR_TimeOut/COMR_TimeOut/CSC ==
  BSWCellBalanceCircuitStatusMsgRx : Inport
  BSWBoardTempMsgRx : Inport  Port=2
  BSWCellTempMsgRx : Inport  Port=3
  BSWCellVoltageMsgRx : Inport  Port=4
  BSWModuleVoltageMsgRx : Inport  Port=5
  DiagEna : Inport  Port=6
  BalCirSta : Stateflow chart  TreatAsAtomicUnit=on
  BoardTmp : Stateflow chart  TreatAsAtomicUnit=on
  CellTmp : Stateflow chart  TreatAsAtomicUnit=on
  CellVol : Stateflow chart  TreatAsAtomicUnit=on
  Constant{1..6} (6 alike) : Constant  Value=COMR_tiCSCMsgTmt_C
  Constant10 : Constant  Value=COMR_UAESFltDiagDisbl_C
  DSM_ReportCheck : Subsystem  TreatAsAtomicUnit=on  RTWFcnName=DSM_ReportCheck  RTWFileName=SrvLib
  DSM_ReportCheck1 : Subsystem  TreatAsAtomicUnit=on  RTWFcnName=DSM_ReportCheck  RTWFileName=SrvLib
  DSM_ReportCheck2 : Subsystem  TreatAsAtomicUnit=on  RTWFcnName=DSM_ReportCheck  RTWFileName=SrvLib
  Data Store Read : DataStoreRead  DataStoreName=DFC_BoardTempTmt
  Data Store Read1 : DataStoreRead  DataStoreName=DFC_CellTempTmt
  Data Store Read2 : DataStoreRead  DataStoreName=DFC_CellVoltTmt
  Data Store Write : DataStoreWrite  DataStoreName=DFC_BoardTempTmt
  Data Store Write1 : DataStoreWrite  DataStoreName=DFC_CellTempTmt
  Data Store Write2 : DataStoreWrite  DataStoreName=DFC_CellVoltTmt
  Logical Operator{1,3..5,7,11} (6 alike) : Logic  Operator=NOT  AllPortsSameDT=off  OutDataTypeStr=boolean
  Logical Operator10 : Logic  Operator=OR  AllPortsSameDT=off  OutDataTypeStr=boolean
  Logical Operator12 : Logic  Operator=OR  AllPortsSameDT=off  OutDataTypeStr=boolean
  Logical Operator2 : Logic  Inputs=3  AllPortsSameDT=off  OutDataTypeStr=boolean
  Logical Operator6 : Logic  Inputs=3  AllPortsSameDT=off  OutDataTypeStr=boolean
  Logical Operator8 : Logic  Operator=OR  AllPortsSameDT=off  OutDataTypeStr=boolean
  Logical Operator9 : Logic  Inputs=3  AllPortsSameDT=off  OutDataTypeStr=boolean
  ModuVol : Stateflow chart  TreatAsAtomicUnit=on
  TONV_10msTimeDebounce1 : Subsystem  TreatAsAtomicUnit=on  RTWFcnName=TONV_10msTimeDebounce  RTWFileName=SrvLib
  TONV_10msTimeDebounce2 : Subsystem  TreatAsAtomicUnit=on  RTWFcnName=TONV_10msTimeDebounce  RTWFileName=SrvLib
  TONV_10msTimeDebounce3 : Subsystem  TreatAsAtomicUnit=on  RTWFcnName=TONV_10msTimeDebounce  RTWFileName=SrvLib
  TONV_10msTimeDebounce4 : Subsystem  TreatAsAtomicUnit=on  RTWFcnName=TONV_10msTimeDebounce  RTWFileName=SrvLib
  TONV_10msTimeDebounce5 : Subsystem  TreatAsAtomicUnit=on  RTWFcnName=TONV_10msTimeDebounce  RTWFileName=SrvLib
  TONV_10msTimeDebounce6 : Subsystem  TreatAsAtomicUnit=on  RTWFcnName=TONV_10msTimeDebounce  RTWFileName=SrvLib
  COMR_flgTmtBalCirSta : Outport
  COMR_flgTmtModuVol : Outport  Port=2
  COMR_bTmtBoardTmpDet : Outport  Port=3
  COMR_bTmtBoardTmpHeal : Outport  Port=4
  COMR_bTmtCellTmpDet : Outport  Port=5
  COMR_bTmtCellTmpHeal : Outport  Port=6
  COMR_bTmtCellVolDet : Outport  Port=7
  COMR_bTmtCellVolHeal : Outport  Port=8
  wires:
  BalCirSta/1(COMR_flgTmtBalCirSta) -> COMR_flgTmtBalCirSta/1
  BSWCellBalanceCircuitStatusMsgRx/1 -> BalCirSta/1(BSWCellBalanceCircuitStatusMsgRx)
  BSWBoardTempMsgRx/1 -> BoardTmp/1(BSWBoardTempMsgRx)
  BSWCellTempMsgRx/1 -> CellTmp/1(BSWCellTempMsgRx)
  BSWCellVoltageMsgRx/1 -> CellVol/1(BSWCellVoltageMsgRx)
  BSWModuleVoltageMsgRx/1 -> ModuVol/1(BSWModuleVoltageMsgRx)
  ModuVol/1(COMR_flgTmtModuVol) -> COMR_flgTmtModuVol/1
  CellTmp/1(COMR_flgTmtCellTmp) -> Logical Operator2/2, Logical Operator3/1
  Constant4/1 -> TONV_10msTimeDebounce6/2(T)
  CellVol/1(COMR_flgTmtCellVol) -> Logical Operator6/2, Logical Operator1/1
  Constant1/1 -> TONV_10msTimeDebounce1/2(T)
  BoardTmp/1(COMR_flgTmtBoardTmp) -> Logical Operator9/2, Logical Operator4/1
  Constant2/1 -> TONV_10msTimeDebounce2/2(T)
  TONV_10msTimeDebounce2/1(y) -> DSM_ReportCheck/2(Err), COMR_bTmtBoardTmpDet/1
  Constant3/1 -> TONV_10msTimeDebounce3/2(T)
  TONV_10msTimeDebounce3/1(y) -> DSM_ReportCheck/3(Heal), COMR_bTmtBoardTmpHeal/1
  Constant5/1 -> TONV_10msTimeDebounce4/2(T)
  TONV_10msTimeDebounce4/1(y) -> DSM_ReportCheck1/3(Heal), COMR_bTmtCellTmpHeal/1
  Constant6/1 -> TONV_10msTimeDebounce5/2(T)
  TONV_10msTimeDebounce5/1(y) -> DSM_ReportCheck2/3(Heal), COMR_bTmtCellVolHeal/1
  DSM_ReportCheck/1(Dfc_id) -> Data Store Write/1
  Data Store Read/1 -> DSM_ReportCheck/1(Dfc_id_nv)
  Data Store Read1/1 -> DSM_ReportCheck1/1(Dfc_id_nv)
  DSM_ReportCheck1/1(Dfc_id) -> Data Store Write1/1
  DSM_ReportCheck2/1(Dfc_id) -> Data Store Write2/1
  Data Store Read2/1 -> DSM_ReportCheck2/1(Dfc_id_nv)
  Logical Operator4/1 -> Logical Operator8/2
  Logical Operator1/1 -> Logical Operator12/2
  Logical Operator3/1 -> Logical Operator10/2
  TONV_10msTimeDebounce6/1(y) -> DSM_ReportCheck1/2(Err), COMR_bTmtCellTmpDet/1
  TONV_10msTimeDebounce1/1(y) -> DSM_ReportCheck2/2(Err), COMR_bTmtCellVolDet/1
  DiagEna/1 -> Logical Operator9/1, Logical Operator2/1, Logical Operator6/1
  Logical Operator9/1 -> TONV_10msTimeDebounce2/1(u)
  Logical Operator2/1 -> TONV_10msTimeDebounce6/1(u)
  Logical Operator6/1 -> TONV_10msTimeDebounce1/1(u)
  Logical Operator7/1 -> Logical Operator9/3
  Constant10/1 -> Logical Operator7/1, Logical Operator8/1, Logical Operator5/1, Logical Operator10/1, Logical Operator11/1, Logical Operator12/1
  Logical Operator8/1 -> TONV_10msTimeDebounce3/1(u)
  Logical Operator5/1 -> Logical Operator2/3
  Logical Operator10/1 -> TONV_10msTimeDebounce4/1(u)
  Logical Operator11/1 -> Logical Operator6/3
  Logical Operator12/1 -> TONV_10msTimeDebounce5/1(u)

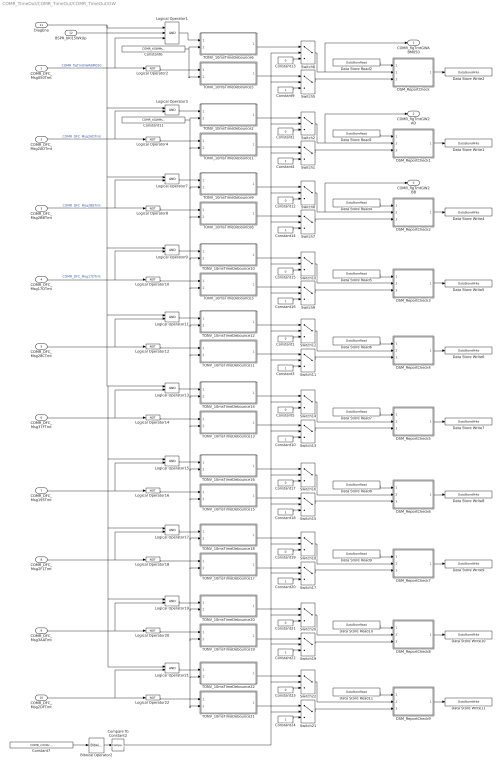
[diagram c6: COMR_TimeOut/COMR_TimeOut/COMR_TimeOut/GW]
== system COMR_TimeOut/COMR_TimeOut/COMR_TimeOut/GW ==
  COMR_DFC_Msg050Tmt : Inport
  COMR_DFC_Msg2ADTmt : Inport  Port=2
  COMR_DFC_Msg2BBTmt : Inport  Port=3
  COMR_DFC_Msg17DTmt : Inport  Port=4
  COMR_DFC_Msg28CTmt : Inport  Port=5
  COMR_DFC_Msg37FTmt : Inport  Port=6
  COMR_DFC_Msg195Tmt : Inport  Port=7
  COMR_DFC_Msg2F1Tmt : Inport  Port=8
  COMR_DFC_Msg3AATmt : Inport  Port=9
  COMR_DFC_Msg2DFTmt : Inport  Port=10
  DiagEna : Inport  Port=11
  BSPR_bKl15WkUp : Inport  Port=12  OutDataTypeStr=boolean
  Bitwise Operator2 : simulink/Logic and Bit Operations/Bitwise Operator  logicop=AND  UseBitMask=on  BitMask=bin2dec('00010000')  BitMaskRealWorld=Stored Integer
  Compare To Constant2 : simulink/Logic and Bit Operations/Compare To Constant  relop===  const=16  OutDataTypeStr=boolean
  Constant{1..2,5,12..13,15,17,19,21,23} (10 alike) : Constant  Value=0  OutDataTypeStr=boolean
  Constant{3..4,9..10,14,16,18,20,22,24} (10 alike) : Constant  OutDataTypeStr=boolean
  Constant11 : Constant  Value=COMR_tiGWMsgTmt_C
  Constant6 : Constant  Value=COMR_tiGWMsg050Tmt_C
  Constant7 : Constant  Value=COMR_cntObcTmtDiag_CW
  DSM_ReportCheck : Subsystem  TreatAsAtomicUnit=on  RTWFcnName=DSM_ReportCheck  RTWFileName=SrvLib
  DSM_ReportCheck1 : Subsystem  TreatAsAtomicUnit=on  RTWFcnName=DSM_ReportCheck  RTWFileName=SrvLib
  DSM_ReportCheck2 : Subsystem  TreatAsAtomicUnit=on  RTWFcnName=DSM_ReportCheck  RTWFileName=SrvLib
  DSM_ReportCheck3 : Subsystem  TreatAsAtomicUnit=on  RTWFcnName=DSM_ReportCheck  RTWFileName=SrvLib
  DSM_ReportCheck4 : Subsystem  TreatAsAtomicUnit=on  RTWFcnName=DSM_ReportCheck  RTWFileName=SrvLib
  DSM_ReportCheck5 : Subsystem  TreatAsAtomicUnit=on  RTWFcnName=DSM_ReportCheck  RTWFileName=SrvLib
  DSM_ReportCheck6 : Subsystem  TreatAsAtomicUnit=on  RTWFcnName=DSM_ReportCheck  RTWFileName=SrvLib
  DSM_ReportCheck7 : Subsystem  TreatAsAtomicUnit=on  RTWFcnName=DSM_ReportCheck  RTWFileName=SrvLib
  DSM_ReportCheck8 : Subsystem  TreatAsAtomicUnit=on  RTWFcnName=DSM_ReportCheck  RTWFileName=SrvLib
  DSM_ReportCheck9 : Subsystem  TreatAsAtomicUnit=on  RTWFcnName=DSM_ReportCheck  RTWFileName=SrvLib
  Data Store Read1 : DataStoreRead  DataStoreName=DFC_Msg2ADTmt
  Data Store Read10 : DataStoreRead  DataStoreName=DFC_Msg3AATmt
  Data Store Read11 : DataStoreRead  DataStoreName=DFC_Msg2DFTmt
  Data Store Read2 : DataStoreRead  DataStoreName=DFC_Msg050Tmt
  Data Store Read4 : DataStoreRead  DataStoreName=DFC_Msg2BBTmt
  Data Store Read5 : DataStoreRead  DataStoreName=DFC_Msg17DTmt
  Data Store Read6 : DataStoreRead  DataStoreName=DFC_Msg28CTmt
  Data Store Read7 : DataStoreRead  DataStoreName=DFC_Msg37FTmt
  Data Store Read8 : DataStoreRead  DataStoreName=DFC_Msg195Tmt
  Data Store Read9 : DataStoreRead  DataStoreName=DFC_Msg2F1Tmt
  Data Store Write1 : DataStoreWrite  DataStoreName=DFC_Msg2ADTmt
  Data Store Write10 : DataStoreWrite  DataStoreName=DFC_Msg3AATmt
  Data Store Write11 : DataStoreWrite  DataStoreName=DFC_Msg2DFTmt
  Data Store Write2 : DataStoreWrite  DataStoreName=DFC_Msg050Tmt
  Data Store Write4 : DataStoreWrite  DataStoreName=DFC_Msg2BBTmt
  Data Store Write5 : DataStoreWrite  DataStoreName=DFC_Msg17DTmt
  Data Store Write6 : DataStoreWrite  DataStoreName=DFC_Msg28CTmt
  Data Store Write7 : DataStoreWrite  DataStoreName=DFC_Msg37FTmt
  Data Store Write8 : DataStoreWrite  DataStoreName=DFC_Msg195Tmt
  Data Store Write9 : DataStoreWrite  DataStoreName=DFC_Msg2F1Tmt
  Logical Operator1 : Logic  Inputs=3  AllPortsSameDT=off  OutDataTypeStr=boolean
  Logical Operator{2,4,8,10,12,14,16,18,20,22} (10 alike) : Logic  Operator=NOT  AllPortsSameDT=off  OutDataTypeStr=boolean
  Logical Operator{3,7,9,11,13,15,17,19,21} (9 alike) : Logic  AllPortsSameDT=off  OutDataTypeStr=boolean
  Switch{1..2,5..22} (20 alike) : Switch  Criteria=u2 > Threshold
  TONV_10msTimeDebounce1 : Subsystem  TreatAsAtomicUnit=on  RTWFcnName=TONV_10msTimeDebounce  RTWFileName=SrvLib
  TONV_10msTimeDebounce10 : Subsystem  TreatAsAtomicUnit=on  RTWFcnName=TONV_10msTimeDebounce  RTWFileName=SrvLib
  TONV_10msTimeDebounce11 : Subsystem  TreatAsAtomicUnit=on  RTWFcnName=TONV_10msTimeDebounce  RTWFileName=SrvLib
  TONV_10msTimeDebounce12 : Subsystem  TreatAsAtomicUnit=on  RTWFcnName=TONV_10msTimeDebounce  RTWFileName=SrvLib
  TONV_10msTimeDebounce13 : Subsystem  TreatAsAtomicUnit=on  RTWFcnName=TONV_10msTimeDebounce  RTWFileName=SrvLib
  TONV_10msTimeDebounce14 : Subsystem  TreatAsAtomicUnit=on  RTWFcnName=TONV_10msTimeDebounce  RTWFileName=SrvLib
  TONV_10msTimeDebounce15 : Subsystem  TreatAsAtomicUnit=on  RTWFcnName=TONV_10msTimeDebounce  RTWFileName=SrvLib
  TONV_10msTimeDebounce16 : Subsystem  TreatAsAtomicUnit=on  RTWFcnName=TONV_10msTimeDebounce  RTWFileName=SrvLib
  TONV_10msTimeDebounce17 : Subsystem  TreatAsAtomicUnit=on  RTWFcnName=TONV_10msTimeDebounce  RTWFileName=SrvLib
  TONV_10msTimeDebounce18 : Subsystem  TreatAsAtomicUnit=on  RTWFcnName=TONV_10msTimeDebounce  RTWFileName=SrvLib
  TONV_10msTimeDebounce19 : Subsystem  TreatAsAtomicUnit=on  RTWFcnName=TONV_10msTimeDebounce  RTWFileName=SrvLib
  TONV_10msTimeDebounce2 : Subsystem  TreatAsAtomicUnit=on  RTWFcnName=TONV_10msTimeDebounce  RTWFileName=SrvLib
  TONV_10msTimeDebounce20 : Subsystem  TreatAsAtomicUnit=on  RTWFcnName=TONV_10msTimeDebounce  RTWFileName=SrvLib
  TONV_10msTimeDebounce21 : Subsystem  TreatAsAtomicUnit=on  RTWFcnName=TONV_10msTimeDebounce  RTWFileName=SrvLib
  TONV_10msTimeDebounce22 : Subsystem  TreatAsAtomicUnit=on  RTWFcnName=TONV_10msTimeDebounce  RTWFileName=SrvLib
  TONV_10msTimeDebounce3 : Subsystem  TreatAsAtomicUnit=on  RTWFcnName=TONV_10msTimeDebounce  RTWFileName=SrvLib
  TONV_10msTimeDebounce5 : Subsystem  TreatAsAtomicUnit=on  RTWFcnName=TONV_10msTimeDebounce  RTWFileName=SrvLib
  TONV_10msTimeDebounce6 : Subsystem  TreatAsAtomicUnit=on  RTWFcnName=TONV_10msTimeDebounce  RTWFileName=SrvLib
  TONV_10msTimeDebounce8 : Subsystem  TreatAsAtomicUnit=on  RTWFcnName=TONV_10msTimeDebounce  RTWFileName=SrvLib
  TONV_10msTimeDebounce9 : Subsystem  TreatAsAtomicUnit=on  RTWFcnName=TONV_10msTimeDebounce  RTWFileName=SrvLib
  COMR_flgTmtGWABM050 : Outport
  COMR_flgTmtGW2AD : Outport  Port=2
  COMR_flgTmtGW2BB : Outport  Port=3
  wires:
  Logical Operator2/1 -> TONV_10msTimeDebounce5/1(u)
  Logical Operator1/1 -> TONV_10msTimeDebounce6/1(u)
  COMR_DFC_Msg050Tmt/1 -> Logical Operator1/3, Logical Operator2/1  "COMR_flgTmtGWABM050"
  Switch6/1 -> DSM_ReportCheck/2(Err), COMR_flgTmtGWABM050/1
  Data Store Read2/1 -> DSM_ReportCheck/1(Dfc_id_nv)
  Switch5/1 -> DSM_ReportCheck/3(Heal)
  TONV_10msTimeDebounce5/1(y) -> Switch5/1
  TONV_10msTimeDebounce6/1(y) -> Switch6/1
  Constant9/1 -> Switch5/3
  Constant13/1 -> Switch6/3
  DSM_ReportCheck/1(Dfc_id) -> Data Store Write2/1
  Bitwise Operator2/1 -> Compare To Constant2/1
  Constant7/1 -> Bitwise Operator2/1
  Compare To Constant2/1 -> Switch21/2, Switch22/2, Switch19/2, Switch20/2, Switch17/2, Switch18/2, Switch15/2, Switch16/2, Switch13/2, Switch14/2, Switch11/2, Switch12/2, Switch9/2, Switch10/2, Switch7/2, Switch8/2, Switch1/2, Switch2/2, Switch6/2, Switch5/2
  Logical Operator4/1 -> TONV_10msTimeDebounce1/1(u)
  Logical Operator3/1 -> TONV_10msTimeDebounce2/1(u)
  COMR_DFC_Msg2ADTmt/1 -> Logical Operator3/2, Logical Operator4/1  "COMR_DFC_Msg2ADTmt"
  Switch2/1 -> DSM_ReportCheck1/2(Err), COMR_flgTmtGW2AD/1
  Data Store Read1/1 -> DSM_ReportCheck1/1(Dfc_id_nv)
  Switch1/1 -> DSM_ReportCheck1/3(Heal)
  TONV_10msTimeDebounce1/1(y) -> Switch1/1
  TONV_10msTimeDebounce2/1(y) -> Switch2/1
  Constant4/1 -> Switch1/3
  Constant2/1 -> Switch2/3
  DSM_ReportCheck1/1(Dfc_id) -> Data Store Write1/1
  Logical Operator8/1 -> TONV_10msTimeDebounce8/1(u)
  Logical Operator7/1 -> TONV_10msTimeDebounce9/1(u)
  COMR_DFC_Msg2BBTmt/1 -> Logical Operator7/2, Logical Operator8/1  "COMR_DFC_Msg2BBTmt"
  Switch8/1 -> DSM_ReportCheck2/2(Err), COMR_flgTmtGW2BB/1
  Data Store Read4/1 -> DSM_ReportCheck2/1(Dfc_id_nv)
  Switch7/1 -> DSM_ReportCheck2/3(Heal)
  TONV_10msTimeDebounce8/1(y) -> Switch7/1
  TONV_10msTimeDebounce9/1(y) -> Switch8/1
  Constant14/1 -> Switch7/3
  Constant12/1 -> Switch8/3
  DSM_ReportCheck2/1(Dfc_id) -> Data Store Write4/1
  Logical Operator10/1 -> TONV_10msTimeDebounce3/1(u)
  Logical Operator9/1 -> TONV_10msTimeDebounce10/1(u)
  COMR_DFC_Msg17DTmt/1 -> Logical Operator9/2, Logical Operator10/1  "COMR_DFC_Msg17DTmt"
  Switch10/1 -> DSM_ReportCheck3/2(Err)
  Data Store Read5/1 -> DSM_ReportCheck3/1(Dfc_id_nv)
  Switch9/1 -> DSM_ReportCheck3/3(Heal)
  TONV_10msTimeDebounce3/1(y) -> Switch9/1
  TONV_10msTimeDebounce10/1(y) -> Switch10/1
  Constant16/1 -> Switch9/3
  Constant15/1 -> Switch10/3
  DSM_ReportCheck3/1(Dfc_id) -> Data Store Write5/1
  Logical Operator12/1 -> TONV_10msTimeDebounce11/1(u)
  Logical Operator11/1 -> TONV_10msTimeDebounce12/1(u)
  COMR_DFC_Msg28CTmt/1 -> Logical Operator11/2, Logical Operator12/1
  Switch12/1 -> DSM_ReportCheck4/2(Err)
  Data Store Read6/1 -> DSM_ReportCheck4/1(Dfc_id_nv)
  Switch11/1 -> DSM_ReportCheck4/3(Heal)
  TONV_10msTimeDebounce11/1(y) -> Switch11/1
  TONV_10msTimeDebounce12/1(y) -> Switch12/1
  Constant3/1 -> Switch11/3
  Constant1/1 -> Switch12/3
  DSM_ReportCheck4/1(Dfc_id) -> Data Store Write6/1
  Logical Operator14/1 -> TONV_10msTimeDebounce13/1(u)
  Logical Operator13/1 -> TONV_10msTimeDebounce14/1(u)
  COMR_DFC_Msg37FTmt/1 -> Logical Operator13/2, Logical Operator14/1
  Switch14/1 -> DSM_ReportCheck5/2(Err)
  Data Store Read7/1 -> DSM_ReportCheck5/1(Dfc_id_nv)
  Switch13/1 -> DSM_ReportCheck5/3(Heal)
  TONV_10msTimeDebounce13/1(y) -> Switch13/1
  TONV_10msTimeDebounce14/1(y) -> Switch14/1
  Constant10/1 -> Switch13/3
  Constant5/1 -> Switch14/3
  DSM_ReportCheck5/1(Dfc_id) -> Data Store Write7/1
  Logical Operator16/1 -> TONV_10msTimeDebounce15/1(u)
  Logical Operator15/1 -> TONV_10msTimeDebounce16/1(u)
  COMR_DFC_Msg195Tmt/1 -> Logical Operator15/2, Logical Operator16/1
  Switch16/1 -> DSM_ReportCheck6/2(Err)
  Data Store Read8/1 -> DSM_ReportCheck6/1(Dfc_id_nv)
  Switch15/1 -> DSM_ReportCheck6/3(Heal)
  TONV_10msTimeDebounce15/1(y) -> Switch15/1
  TONV_10msTimeDebounce16/1(y) -> Switch16/1
  Constant18/1 -> Switch15/3
  Constant17/1 -> Switch16/3
  DSM_ReportCheck6/1(Dfc_id) -> Data Store Write8/1
  Logical Operator18/1 -> TONV_10msTimeDebounce17/1(u)
  Logical Operator17/1 -> TONV_10msTimeDebounce18/1(u)
  COMR_DFC_Msg2F1Tmt/1 -> Logical Operator17/2, Logical Operator18/1
  Switch18/1 -> DSM_ReportCheck7/2(Err)
  Data Store Read9/1 -> DSM_ReportCheck7/1(Dfc_id_nv)
  Switch17/1 -> DSM_ReportCheck7/3(Heal)
  TONV_10msTimeDebounce17/1(y) -> Switch17/1
  TONV_10msTimeDebounce18/1(y) -> Switch18/1
  Constant20/1 -> Switch17/3
  Constant19/1 -> Switch18/3
  DSM_ReportCheck7/1(Dfc_id) -> Data Store Write9/1
  Logical Operator20/1 -> TONV_10msTimeDebounce19/1(u)
  Logical Operator19/1 -> TONV_10msTimeDebounce20/1(u)
  COMR_DFC_Msg3AATmt/1 -> Logical Operator19/2, Logical Operator20/1
  Switch20/1 -> DSM_ReportCheck8/2(Err)
  Data Store Read10/1 -> DSM_ReportCheck8/1(Dfc_id_nv)
  Switch19/1 -> DSM_ReportCheck8/3(Heal)
  TONV_10msTimeDebounce19/1(y) -> Switch19/1
  TONV_10msTimeDebounce20/1(y) -> Switch20/1
  Constant22/1 -> Switch19/3
  Constant21/1 -> Switch20/3
  DSM_ReportCheck8/1(Dfc_id) -> Data Store Write10/1
  Logical Operator22/1 -> TONV_10msTimeDebounce21/1(u)
  Logical Operator21/1 -> TONV_10msTimeDebounce22/1(u)
  COMR_DFC_Msg2DFTmt/1 -> Logical Operator21/2, Logical Operator22/1
  Switch22/1 -> DSM_ReportCheck9/2(Err)
  Data Store Read11/1 -> DSM_ReportCheck9/1(Dfc_id_nv)
  Switch21/1 -> DSM_ReportCheck9/3(Heal)
  TONV_10msTimeDebounce21/1(y) -> Switch21/1
  TONV_10msTimeDebounce22/1(y) -> Switch22/1
  Constant24/1 -> Switch21/3
  Constant23/1 -> Switch22/3
  Constant11/1 -> TONV_10msTimeDebounce21/2(T), TONV_10msTimeDebounce22/2(T), TONV_10msTimeDebounce19/2(T), TONV_10msTimeDebounce20/2(T), TONV_10msTimeDebounce17/2(T), TONV_10msTimeDebounce18/2(T), TONV_10msTimeDebounce15/2(T), TONV_10msTimeDebounce16/2(T), TONV_10msTimeDebounce13/2(T), TONV_10msTimeDebounce14/2(T), TONV_10msTimeDebounce11/2(T), TONV_10msTimeDebounce12/2(T), TONV_10msTimeDebounce3/2(T), TONV_10msTimeDebounce10/2(T), TONV_10msTimeDebounce8/2(T), TONV_10msTimeDebounce9/2(T), TONV_10msTimeDebounce1/2(T), TONV_10msTimeDebounce2/2(T)
  DSM_ReportCheck9/1(Dfc_id) -> Data Store Write11/1
  DiagEna/1 -> Logical Operator21/1, Logical Operator19/1, Logical Operator17/1, Logical Operator15/1, Logical Operator13/1, Logical Operator11/1, Logical Operator9/1, Logical Operator7/1, Logical Operator3/1, Logical Operator1/1
  BSPR_bKl15WkUp/1 -> Logical Operator1/2
  Constant6/1 -> TONV_10msTimeDebounce5/2(T), TONV_10msTimeDebounce6/2(T)

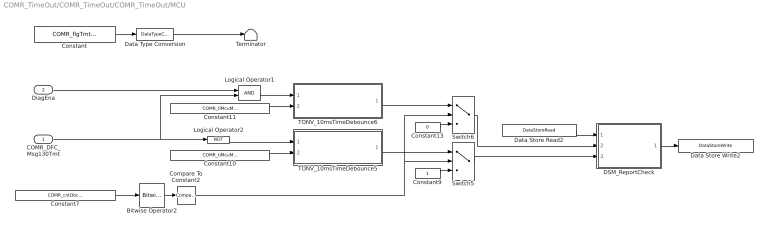
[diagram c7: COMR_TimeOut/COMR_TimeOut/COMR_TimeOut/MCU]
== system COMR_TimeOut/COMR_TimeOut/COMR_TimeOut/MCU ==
  COMR_DFC_Msg130Tmt : Inport
  DiagEna : Inport  Port=2
  Bitwise Operator2 : simulink/Logic and Bit Operations/Bitwise Operator  logicop=AND  UseBitMask=on  BitMask=bin2dec('00010000')  BitMaskRealWorld=Stored Integer
  Compare To Constant2 : simulink/Logic and Bit Operations/Compare To Constant  relop===  const=16  OutDataTypeStr=boolean
  Constant : Constant  Value=COMR_flgTmtCAB_C
  Constant10 : Constant  Value=COMR_tiMcuMsgTmt_C
  Constant11 : Constant  Value=COMR_tiMcuMsgTmt_C
  Constant13 : Constant  Value=0  OutDataTypeStr=boolean
  Constant7 : Constant  Value=COMR_cntObcTmtDiag_CW
  Constant9 : Constant  OutDataTypeStr=boolean
  DSM_ReportCheck : Subsystem  TreatAsAtomicUnit=on  RTWFcnName=DSM_ReportCheck  RTWFileName=SrvLib
  Data Store Read2 : DataStoreRead  DataStoreName=DFC_Msg130Tmt
  Data Store Write2 : DataStoreWrite  DataStoreName=DFC_Msg130Tmt
  Data Type Conversion : DataTypeConversion  OutDataTypeStr=boolean
  Logical Operator1 : Logic  AllPortsSameDT=off  OutDataTypeStr=boolean
  Logical Operator2 : Logic  Operator=NOT  AllPortsSameDT=off  OutDataTypeStr=boolean
  Switch5 : Switch  Criteria=u2 > Threshold
  Switch6 : Switch  Criteria=u2 > Threshold
  TONV_10msTimeDebounce5 : Subsystem  TreatAsAtomicUnit=on  RTWFcnName=TONV_10msTimeDebounce  RTWFileName=SrvLib
  TONV_10msTimeDebounce6 : Subsystem  TreatAsAtomicUnit=on  RTWFcnName=TONV_10msTimeDebounce  RTWFileName=SrvLib
  Terminator : Terminator
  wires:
  Logical Operator2/1 -> TONV_10msTimeDebounce5/1(u)
  Logical Operator1/1 -> TONV_10msTimeDebounce6/1(u)
  COMR_DFC_Msg130Tmt/1 -> Logical Operator1/2, Logical Operator2/1
  Switch6/1 -> DSM_ReportCheck/2(Err)
  Data Store Read2/1 -> DSM_ReportCheck/1(Dfc_id_nv)
  Switch5/1 -> DSM_ReportCheck/3(Heal)
  TONV_10msTimeDebounce5/1(y) -> Switch5/1
  TONV_10msTimeDebounce6/1(y) -> Switch6/1
  Constant9/1 -> Switch5/3
  Constant13/1 -> Switch6/3
  Constant10/1 -> TONV_10msTimeDebounce5/2(T)
  DSM_ReportCheck/1(Dfc_id) -> Data Store Write2/1
  Constant11/1 -> TONV_10msTimeDebounce6/2(T)
  DiagEna/1 -> Logical Operator1/1
  Bitwise Operator2/1 -> Compare To Constant2/1
  Constant7/1 -> Bitwise Operator2/1
  Compare To Constant2/1 -> Switch6/2, Switch5/2
  Data Type Conversion/1 -> Terminator/1
  Constant/1 -> Data Type Conversion/1
